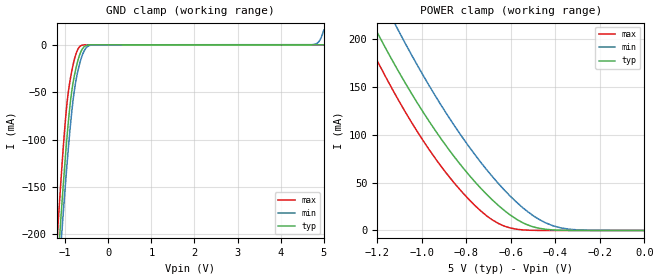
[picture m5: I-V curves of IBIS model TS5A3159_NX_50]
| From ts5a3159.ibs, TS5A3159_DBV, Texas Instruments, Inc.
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[Model]   TS5A3159_NX_50
Model_type  Terminator
| variable   typ   min   max
C_comp   23.49pF   20.86pF   24.52pF
| C_tri-state   23.49pF   20.86pF   24.52pF
[Temperature Range]   40   100   -40
| Ambient temperature   25   85   -40
[Voltage range]   5   4.5   5.5
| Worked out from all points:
|   GND clamp passes 1 mA (typ) near -0.52 V on its own axis
|   POWER clamp passes 1 mA (typ) near -0.43 V on its own axis
[GND Clamp]
| TS5A3159_NX_50
|   Voltage   I(typ)   I(min)   I(max)
-5V       -3.911A    -3.755A    -4.165A
-1.2V     -251.8mA   -279.4mA   -215.7mA
-1.165V   -227.4mA   -255.7mA   -190.1mA
-1.13V    -203.6mA   -232.5mA   -165.3mA
-1.07V    -164.4mA   -193.9mA   -124.9mA
-925mV    -80.96mA   -108.7mA   -49.4mA
-790mV    -33.51mA   -49.32mA   -16.16mA
-625mV    -6.383mA   -13.94mA   -758.2uA
-390mV    -28.86uA   -271.6uA   -169nA
4.73V     239.2pA    128uA      101.5pA
4.885V    266.8pA    3.207mA    106.7pA
5V        1.607nA    15.56mA    110.6pA
[POWER Clamp]
| TS5A3159_NX_50
|   Voltage   I(typ)   I(min)   I(max)
-5V       3.281A     3.376A     3.507A
-1.285V   246mA      294.6mA    217.7mA
-1.255V   231.9mA    279.6mA    203.1mA
-1.195V   204.8mA    250.5mA    175.2mA
-1.105V   166.6mA    209.2mA    136.5mA
-935mV    103.2mA    139.2mA    74.07mA
-790mV    58.62mA    88.38mA    32.93mA
-655mV    26.01mA    48.91mA    7.266mA
-530mV    6.362mA    20.74mA    382.3uA
-445mV    1.258mA    8.112mA    23uA
-375mV    233uA      2.688mA    1.585uA
0V        0A         0A         0A
